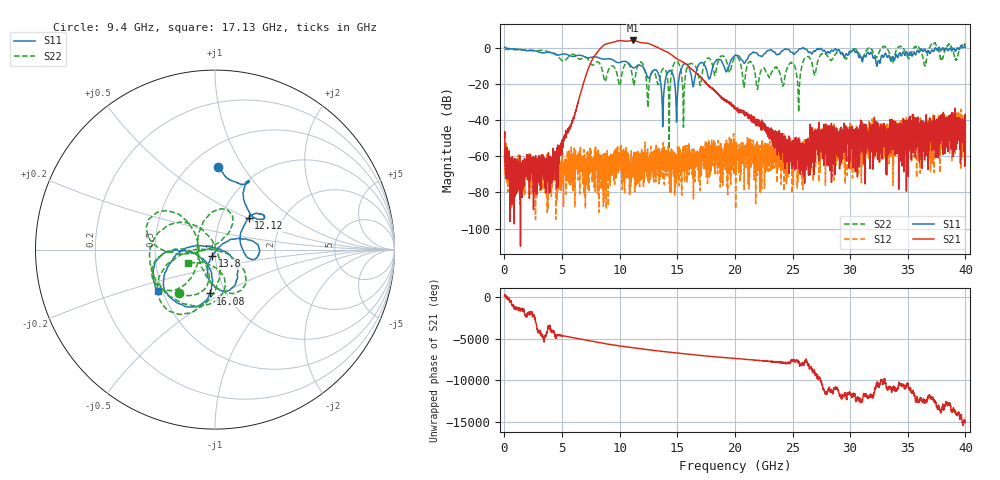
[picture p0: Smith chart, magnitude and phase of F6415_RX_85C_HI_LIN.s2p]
!Keysight Technologies,N5245B,MY52451815,A.15.70.20
!Date: Wednesday, April 17, 2024 16:17:40
!Correction: S33(C  2-Port  )
!S43(C  2-Port  )
!S34(C  2-Port  )
!S44(C  2-Port  )
!S2P File: Measurements: S33, S43, S34, S44:
# Hz S  RI  R 50
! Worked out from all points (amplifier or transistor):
!   4000 points, 10 MHz to 40 GHz, reference 50 ohm
!   highest |S21| = 4.1 dB at 11.15 GHz (marker M1)
!   |S21| within 3 dB of that: 8.54 GHz to 12.99 GHz (4.448 GHz wide, 41.3 % of centre)
!   unconditionally stable (mu >= 1): 99.56 MHz to 25.86 GHz; 25.96 GHz to 32.71 GHz; 34.55 GHz to 35.54 GHz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
!   at 6.67 GHz: K = 6171.10, MAG = -20.3 dB, |S12| = -64.9 dB
!   at 20.01 GHz: K = 4766.78, MAG = -30.1 dB, |S12| = -53.1 dB
!   at 40 GHz: K = 3261.80, MSG = -10.5 dB, |S12| = -41.9 dB
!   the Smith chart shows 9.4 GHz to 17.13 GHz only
!   S11 on the Smith chart (normalised r, x): 9.4 GHz: 0.66, +0.78; 12.12 GHz: 1.35, +0.51; 13.8 GHz: 0.97, -0.07; 16.08 GHz: 0.84, -0.44; 17.13 GHz: 0.47, -0.26
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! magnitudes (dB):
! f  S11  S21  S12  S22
! 10 MHz  0.4  -49.4  -62.9  -0.8
! 1.08 GHz  -0.6  -77.0  -63.9  -1.0
! 3.97 GHz  -2.5  -71.7  -69.6  -2.6
! 6.68 GHz  -4.3  -23.3  -68.3  -6.0
! 9.4 GHz  -6.7  3.1  -65.9  -10.0
! 11.15 GHz  -10.9  4.1  -60.6  -18.1
! 12.12 GHz  -11.8  2.7  -74.1  -10.7
! 13.34 GHz  -14.1  0.1  -61.2  -20.1
! 13.8 GHz  -28.0  -1.4  -65.2  -11.5
! 14.33 GHz  -12.5  -3.0  -59.1  -28.9
! 15.01 GHz  -26.1  -6.3  -60.6  -7.6
! 15.55 GHz  -9.0  -8.1  -63.7  -33.8
! 16.08 GHz  -12.2  -10.8  -65.0  -8.7
! 17.13 GHz  -8.1  -16.8  -61.2  -15.4
! 20.01 GHz  -4.1  -33.8  -53.1  -5.3
! 21.96 GHz  -3.2  -43.2  -58.5  -23.0
! 25.52 GHz  -1.1  -60.4  -61.3  -35.3
! 25.86 GHz  0.0  -52.6  -55.4  -8.5
! 26.67 GHz  -3.3  -44.1  -52.1  -8.3
! 33.34 GHz  -4.2  -50.4  -54.5  -1.8
! 39.22 GHz  -1.0  -41.6  -45.6  -6.6
! 40 GHz  0.3  -62.9  -41.9  1.7
